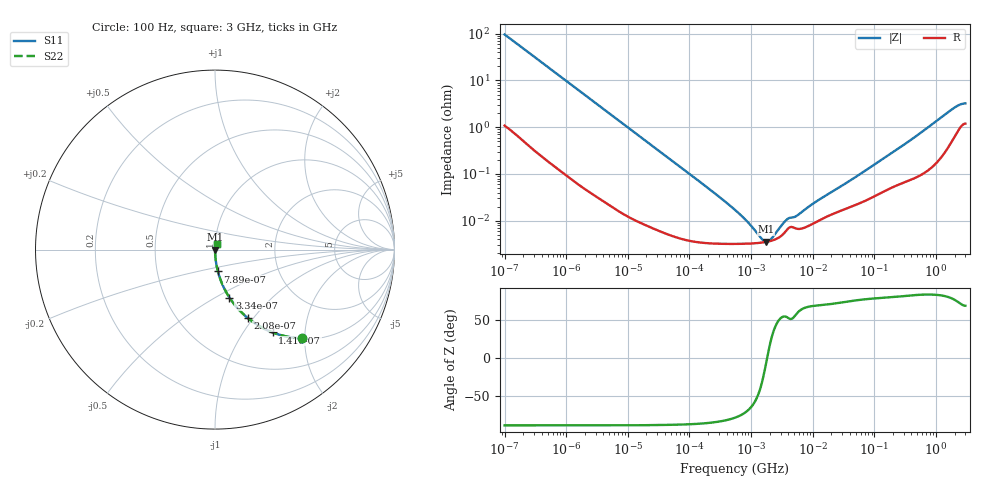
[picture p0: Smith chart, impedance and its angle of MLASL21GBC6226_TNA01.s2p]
! MLASL21GBC6226_TNA01  S-PARAMETER MODEL  ( Standard Model )
! Model Generated by TAIYO YUDEN Corporation (http://www.ty-top.com)
! Version 2.0
! TAIYO YUDEN Control No. 240306
! Copyright(c) 2013 TAIYO YUDEN CO.,LTD. All Rights Reserved.
! Product Description (link to TY-COMPAS)
! https://ds.yuden.co.jp/TYCOMPAS/or/detail?pn=MLASL21GBC6226MTNA01&u=M
! Products Name : Multilayer Ceramic Capacitors
! Characteristics :
!  Capacitance : 22 [uF] , Rated Voltage : 10 [V] , TCC : X6S
!  Case Size : 2.0 x 1.25 / 0.079 x 0.049 [mm/inch] , Thickness : 1.25 / 0.049 [mm/inch]
!  (Conditions: Temperature = 25 [degC] , DC Bias Voltage = 0 [V])
! External Node Assignments :
!  1  o---| |---o  2
! GND o---------o GND
! Frequency Range : 100Hz  -  3GHz  [ 401 STEP ]
# MHZ S RI R 50
! Freq[MHz].  S11 Real  S11 Imag  S21 Real  S21 Imag  S12 Real  S12 Imag  S22 Real  S22 Imag
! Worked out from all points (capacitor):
!   401 points, 100 Hz to 3 GHz, reference 50 ohm
!   read as one part in series: C = 16.5 uF near 109 Hz
!   lowest |Z| = 3.55 mohm at 1.751 MHz (marker M1)
!   series resonance near 1.825 MHz, so ESL is about 460 pH
!   S11 on the Smith chart (normalised r, x): 100 Hz: 1.02, -1.93; 141 Hz: 1.02, -1.37; 208 Hz: 1.01, -0.93; 334 Hz: 1.01, -0.58; 789 Hz: 1.00, -0.25; 3 GHz: 1.02, +0.06
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0.0001  0.482 -0.4941  0.518 0.4941  0.518 0.4941  0.482 -0.4941
0.000141  0.3215 -0.4616  0.6785 0.4616  0.6785 0.4616  0.3215 -0.4616
0.000208  0.1814 -0.3802  0.8186 0.3802  0.8186 0.3802  0.1814 -0.3802
0.000334  0.0805 -0.2673  0.9195 0.2673  0.9195 0.2673  0.0805 -0.2673
0.000789  0.0162 -0.1217  0.9838 0.1217  0.9838 0.1217  0.0162 -0.1217
0.001788  0.00353 -0.0547  0.9965 0.0547  0.9965 0.0547  0.00353 -0.0547
0.005476  0.000524 -0.018  0.9995 0.018  0.9995 0.018  0.000524 -0.018
0.031977  7.03e-05 -0.00312  0.9999 0.00312  0.9999 0.00312  7.03e-05 -0.00312
0.221826  3.29e-05 -0.000448  1 0.000448  1 0.000448  3.29e-05 -0.000448
0.547723  3.19e-05 -0.000168  1 0.000168  1 0.000168  3.19e-05 -0.000168
0.772864  3.22e-05 -0.000107  1 0.000107  1 0.000107  3.22e-05 -0.000107
0.87939  3.23e-05 -8.82e-05  1 8.82e-05  1 8.82e-05  3.23e-05 -8.82e-05
1.75092  3.52e-05 -4.61e-06  1 4.61e-06  1 4.61e-06  3.52e-05 -4.61e-06
3.486191  5.55e-05 7.7e-05  0.9999 -7.7e-05  0.9999 -7.7e-05  5.55e-05 7.7e-05
5.361412  6.81e-05 0.000105  0.9999 -0.000105  0.9999 -0.000105  6.81e-05 0.000105
9.794414  8.49e-05 0.000209  0.9999 -0.000209  0.9999 -0.000209  8.49e-05 0.000209
44.18008  0.000205 0.000753  0.9998 -0.000753  0.9998 -0.000753  0.000205 0.000753
175.1444  0.000488 0.00255  0.9995 -0.00255  0.9995 -0.00255  0.000488 0.00255
451.4794  0.000853 0.00607  0.9991 -0.00607  0.9991 -0.00607  0.000853 0.00607
1950.712  0.0065 0.0247  0.9935 -0.0247  0.9935 -0.0247  0.0065 0.0247
2419.119  0.0102 0.0282  0.9898 -0.0282  0.9898 -0.0282  0.0102 0.0282
3000  0.0127 0.0294  0.9873 -0.0294  0.9873 -0.0294  0.0127 0.0294
